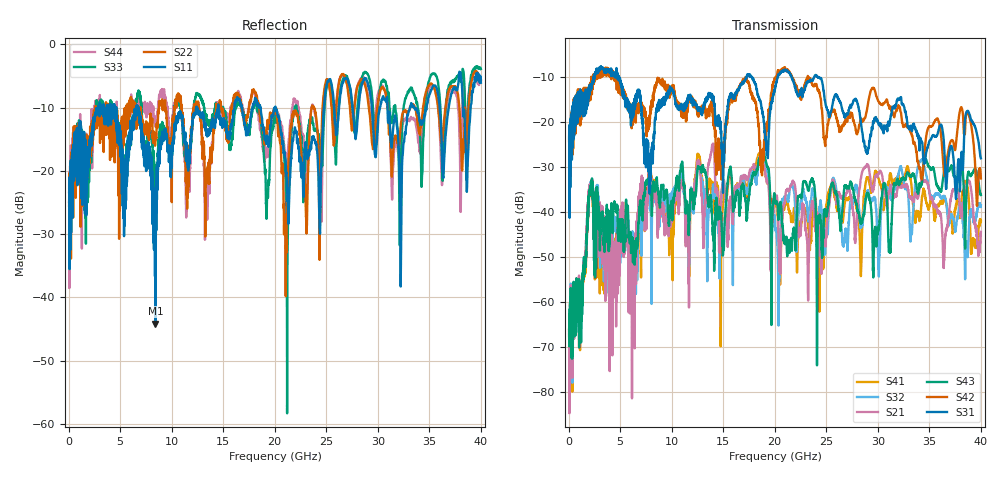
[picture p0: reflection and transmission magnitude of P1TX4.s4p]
!Agilent Technologies,N5245A,MY49151084,A.09.20.08
!Agilent N5245A: A.09.20.08
!Date: Thursday, March 01, 2012 13:14:27
!Correction: S11(Full 4 Port(1,2,3,4))
!S12(Full 4 Port(1,2,3,4))
!S13(Full 4 Port(1,2,3,4))
!S14(Full 4 Port(1,2,3,4))
!S21(Full 4 Port(1,2,3,4))
!S22(Full 4 Port(1,2,3,4))
!S23(Full 4 Port(1,2,3,4))
!S24(Full 4 Port(1,2,3,4))
!S31(Full 4 Port(1,2,3,4))
!S32(Full 4 Port(1,2,3,4))
!S33(Full 4 Port(1,2,3,4))
!S34(Full 4 Port(1,2,3,4))
!S41(Full 4 Port(1,2,3,4))
!S42(Full 4 Port(1,2,3,4))
!S43(Full 4 Port(1,2,3,4))
!S44(Full 4 Port(1,2,3,4))
!S4P File: Measurements: <S11,S12,S13,S14>,
!<S21,S22,S23,S24>,
!<S31,S32,S33,S34>,
!<S41,S42,S43,S44>:
# Hz S  dB  R 50
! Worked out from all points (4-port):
!   3996 points, 50 MHz to 40 GHz, reference 50 ohm
!   strongest paths, dB at 50 MHz, 10.04 GHz, 20.03 GHz, 30.02 GHz, 40 GHz:
!     S31: -23.6, -13.1, -12.6, -19.9, -28.0
!     S42: -24.2, -12.7, -10.3, -15.2, -32.5
!     S43: -66.1, -39.8, -37.3, -44.1, -36.2
!     S21: -67.0, -39.6, -36.7, -31.6, -44.3
!     S32: -67.4, -36.7, -42.2, -48.6, -38.4
!     S41: -65.9, -43.6, -38.1, -32.2, -42.0
!   lowest |S11| = -44.1 dB at 8.43 GHz (marker M1), VSWR 1.01, Z = 50.6 + j0.189 ohm
!   |S11| at or under -10 dB: start of sweep to 2.868 GHz; 6.781 GHz to 12.38 GHz (5.596 GHz wide, 58.4 % of centre); 20.07 GHz to 24.77 GHz (4.692 GHz wide, 20.9 % of centre)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
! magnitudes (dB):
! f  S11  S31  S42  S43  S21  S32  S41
! 50 MHz  -23.4  -23.6  -24.2  -66.1  -67.0  -67.4  -65.9
! 2.14 GHz  -15.1  -12.4  -13.9  -34.7  -33.7  -33.5  -34.8
! 6.13 GHz  -14.2  -17.8  -18.1  -48.7  -55.7  -51.1  -49.6
! 8.43 GHz  -44.1  -19.3  -11.9  -34.8  -35.7  -37.7  -33.9
! 18.77 GHz  -11.7  -17.2  -31.8  -26.8  -28.2  -27.3  -27.7
! 21.03 GHz  -18.1  -8.4  -8.2  -46.5  -36.3  -36.8  -37.9
! 40 GHz  -6.1  -28.0  -32.5  -36.2  -44.3  -38.4  -42.0
